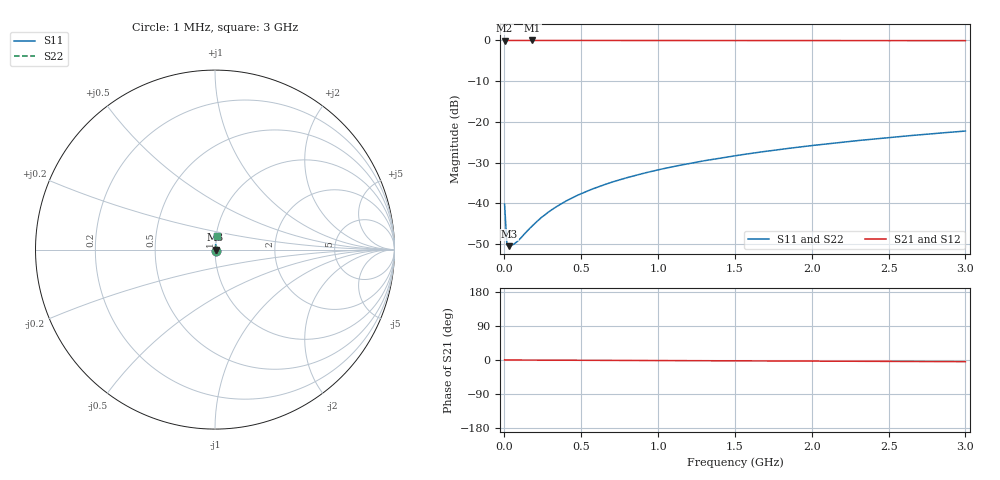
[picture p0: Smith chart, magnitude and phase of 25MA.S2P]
!Keysight Technologies,E4991B,MY54301043,A.02.04
!Date: Thu Nov 16 21:15:10 2023
!Data:
!Freq	S11	S21	S12	S22
# Hz S MA R 50
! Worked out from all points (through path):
!   201 points, 1 MHz to 3 GHz, reference 50 ohm
!   highest |S21| = -0.02 dB at 180.9 MHz (marker M1); lowest = -0.1 dB at 1 MHz (marker M2)
!   lowest |S11| = -50.6 dB at 30.99 MHz (marker M3), VSWR 1.01, Z = 50.3 + j0.0313 ohm
!   |S11| at or under -10 dB: start of sweep to end of sweep
!   |S22| runs from -50.6 to -22.3 dB; largest |S21 - S12| = 0
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1000000  0.009723 -33.5  0.9919 0.3  0.9919 0.3  0.009723 -33.5
1.5995e7  0.003082 -6.2  0.9969 0.0  0.9969 0.0  0.003082 -6.2
3.099e7  0.002968 6.0  0.997 -0.0  0.997 -0.0  0.002968 6.0
4.5985e7  0.003028 15.5  0.9971 -0.0  0.9971 -0.0  0.003028 15.5
7.5975e7  0.003299 30.3  0.9972 -0.1  0.9972 -0.1  0.003299 30.3
1.05965e8  0.003731 41.3  0.9972 -0.1  0.9972 -0.1  0.003731 41.3
1.8094e8  0.005261 58.2  0.9972 -0.3  0.9972 -0.3  0.005261 58.2
2.4092e8  0.006695 65.2  0.9972 -0.3  0.9972 -0.3  0.006695 65.2
3.15895e8  0.008511 70.4  0.9972 -0.5  0.9972 -0.5  0.008511 70.4
4.05865e8  0.01077 74.0  0.9971 -0.6  0.9971 -0.6  0.01077 74.0
5.1083e8  0.01341 76.5  0.997 -0.7  0.997 -0.7  0.01341 76.5
6.15795e8  0.01604 78.2  0.9968 -0.9  0.9968 -0.9  0.01604 78.2
7.05765e8  0.0183 79.1  0.9967 -1.0  0.9967 -1.0  0.0183 79.1
8.55715e8  0.02207 80.2  0.9965 -1.3  0.9965 -1.3  0.02207 80.2
1.005665e9  0.0258 80.9  0.9962 -1.5  0.9962 -1.5  0.0258 80.9
1.125625e9  0.02882 81.4  0.9961 -1.6  0.9961 -1.6  0.02882 81.4
1.275575e9  0.0326 81.7  0.9958 -1.9  0.9958 -1.9  0.0326 81.7
1.5005e9  0.03828 82.0  0.9954 -2.2  0.9954 -2.2  0.03828 82.0
1.725425e9  0.04402 82.2  0.995 -2.5  0.995 -2.5  0.04402 82.2
2.01033e9  0.0513 82.3  0.9944 -2.9  0.9944 -2.9  0.0513 82.3
2.505165e9  0.06408 82.1  0.9932 -3.7  0.9932 -3.7  0.06408 82.1
3e9  0.07695 81.8  0.9919 -4.4  0.9919 -4.4  0.07695 81.8
